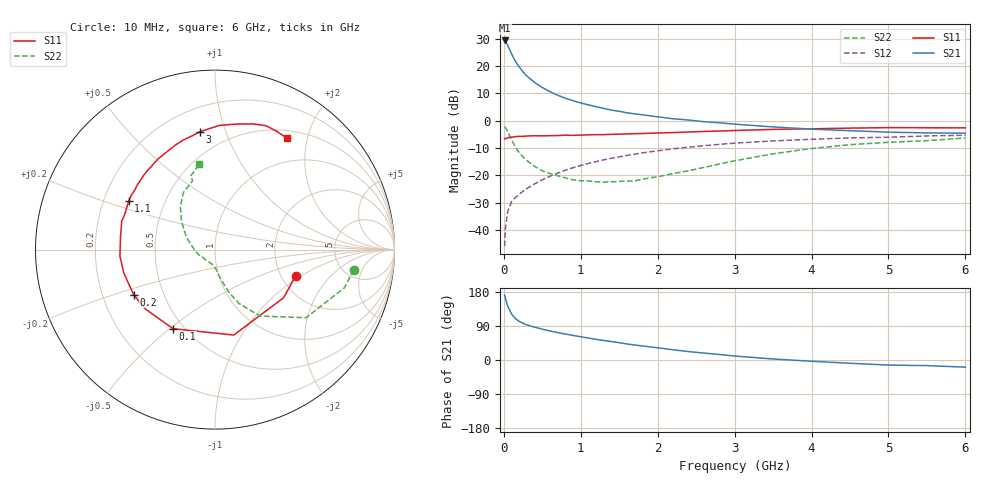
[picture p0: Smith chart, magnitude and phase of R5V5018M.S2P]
! SIEMENS Small Signal Semiconductors
! BFR183
! Si NPN RF Bipolar Junction Transistor in SOT23
! VCE = 0.5 V  IC = 18 mA
! Common Emitter S-Parameters:  May  1996
# GHz  S  MA  R  50
!  f  S11  S21  S12  S22
! GHz  MAG  ANG  MAG  ANG  MAG  ANG  MAG  ANG
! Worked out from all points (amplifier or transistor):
!   36 points, 10 MHz to 6 GHz, reference 50 ohm
!   highest |S21| = 29.3 dB at 10 MHz (marker M1)
!   |S21| within 3 dB of that: start of sweep to 70.1 MHz
!   unconditionally stable (mu >= 1): start of sweep to 10.54 MHz; 272.1 MHz to end of sweep
!   at 250 MHz: K = 0.97, MSG = 21.8 dB, |S12| = -25.8 dB
!   at 1.4 GHz: K = 1.22, MAG = 6.0 dB, |S12| = -13.7 dB
!   at 6 GHz: K = 1.06, MAG = -1.1 dB, |S12| = -5.3 dB
!   S11 on the Smith chart (normalised r, x): 10 MHz: 2.39, -0.90; 100 MHz: 0.44, -0.51; 200 MHz: 0.34, -0.23; 1.1 GHz: 0.31, +0.24; 3 GHz: 0.35, +0.82; 6 GHz: 0.61, +1.66
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0.01  0.4724 -18.1  29.22 171.3  0.0051 79.9  0.7811 -8.3
0.02  0.467 -35.0  28.32 162.8  0.0106 76.0  0.7514 -16.5
0.05  0.4874 -77.6  23.91 142.1  0.022 63.1  0.6335 -36.8
0.1  0.4987 -117.9  16.67 121.3  0.033 54.0  0.4462 -56.0
0.15  0.5104 -139.7  12.2 109.1  0.0396 53.2  0.3293 -65.9
0.2  0.5177 -151.1  9.579 101.9  0.0455 54.9  0.2606 -71.1
0.25  0.5181 -159.8  7.782 96.7  0.0515 56.1  0.2168 -74.3
0.3  0.525 -166.0  6.526 92.7  0.0576 58.2  0.1865 -76.7
0.4  0.5309 -176.1  4.988 86.5  0.0702 60.6  0.1461 -81.5
0.5  0.5281 178.5  4.039 81.4  0.0832 62.0  0.1216 -84.8
0.6  0.5317 172.0  3.388 76.6  0.0967 62.6  0.1082 -87.1
0.7  0.5356 167.1  2.92 72.2  0.1103 62.7  0.0986 -90.8
0.9  0.5398 158.7  2.315 64.8  0.1384 61.9  0.0829 -100.8
1.1  0.5518 150.6  1.943 57.9  0.1658 60.2  0.0795 -110.1
1.3  0.5565 143.4  1.672 51.4  0.1928 57.8  0.0752 -120.5
1.6  0.5741 133.8  1.393 42.3  0.2317 53.9  0.0792 -139.8
2.2  0.6059 116.7  1.085 27.0  0.3063 44.9  0.1081 -173.9
3  0.6617 97.4  0.864 10.5  0.3886 32.1  0.1849 152.8
3.5  0.6927 87.9  0.769 2.7  0.427 24.3  0.2482 139.1
4.5  0.7313 73.3  0.656 -8.6  0.4846 10.5  0.3645 118.7
5.5  0.7431 62.3  0.598 -14.8  0.5263 -0.4  0.4323 108.3
6  0.7394 57.3  0.591 -18.9  0.5414 -7.3  0.4826 100.4
